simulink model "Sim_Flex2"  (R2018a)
settings: Solver=VariableStepAuto  StartTime=0.0  StopTime=20.0  RelTol=1e-3
InitFcn:
  | init
StopFcn:
  | pl
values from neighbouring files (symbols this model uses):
  d2r = 1/r2d    (= 0.0174532925199)    [init.m]
undefined symbols (not defined in the file or in its folder): Af, Ap, Bf, Bp, Cf, Cp, Df, Dp, TVC

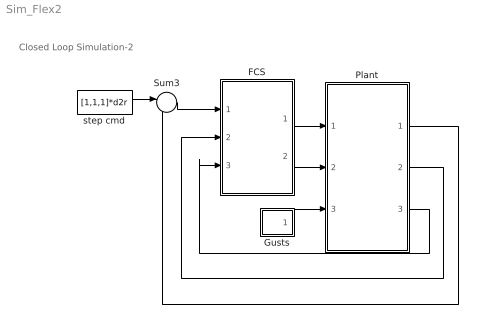
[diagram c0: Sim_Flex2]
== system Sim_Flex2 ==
  note: Closed Loop Simulation-2
  FCS : Subsystem
  Gusts : Subsystem
  Plant : Subsystem
  Sum3 : Sum  Inputs=|-+
  step cmd : Constant  Value=[1,1,1]*d2r
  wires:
  FCS/1(DY) -> Plant/1(Dy)
  FCS/2(DZ) -> Plant/2(Dz)
  Plant/3(NZY) -> FCS/3(Nzy)
  Plant/2(rate) -> FCS/2(pqr)
  Sum3/1 -> FCS/1(Attit)
  Plant/1(attit) -> Sum3/2
  step cmd/1 -> Sum3/1
  Gusts/1(Wgst) -> Plant/3(Gust)

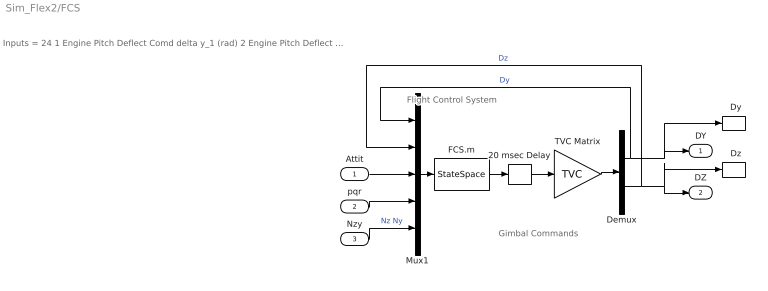
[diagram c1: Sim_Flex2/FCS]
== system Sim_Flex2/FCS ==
  note: Gimbal Commands
  note: Flight Control System
  note: Inputs = 24 1 Engine Pitch Deflect Comd delta y_1 (rad) 2 Engine Pitch Deflect Comd delta y_2 (rad) 3 Engine Pitch Deflect Comd delta y_3 (rad) 4 Engine Pitch Deflect Comd delta y_4 (rad) 5 Engine Pitch Deflect Comd delta y_5 (rad) 6 Engine Pitch Deflect Comd delta y_6 (rad) 7 Engine Pitch Deflect Comd delta y_7 (rad) 8 Engine Pitch Deflect Comd delta y_8 (rad) 9 Engine Yaw Deflect Commnd delta z_1 (rad) 10 Engine Yaw Deflect Commnd delta z_2 (rad) 11 Engine Yaw Deflect Commnd delta z_3 (rad) 12 Engine Yaw Deflect Commnd delta z_4 (rad) 13 Engine Yaw Deflect Commnd delta z_5 (rad) 14 Engine Yaw Deflect Commnd delta z_6 (rad) 15 Engine Yaw Deflect Commnd delta z_7 (rad) 16 Engine Yaw Deflect Commnd delta z_8 (rad) 17 Roll Attitude Error (rad) 18 Pitch Attitude Error (rad) 19 Yaw Attitude Error (rad) 20 Roll Rate (rad/sec) 21 Pitch Rate (rad/sec) 22 Yaw Rate (rad/sec) 23 Normal Acceleration NZ (ft/sec^2) 24 Lateral Acceleration NY (ft/sec^2)
  Attit : Inport
  pqr : Inport  Port=2
  Nzy : Inport  Port=3
  "  Dy" : ToWorkspace  VariableName=DY  SampleTime=-1
  "  Dz" : ToWorkspace  VariableName=DZ  SampleTime=-1
  20 msec Delay : TransportDelay  DelayTime="[1  1  1]*0.02"  InitialOutput="[0  0  0]"  PadeOrder=2
  Demux : Demux  Outputs=[8, 8]
  FCS.m : StateSpace  A=Af  B=Bf  C=Cf  D=Df  InitialCondition=0
  Mux1 : Mux  Inputs=[8, 8, 3, 3, 2]
  TVC Matrix : Gain  Gain=TVC  Multiplication=Matrix(K*u)
  DY : Outport
  DZ : Outport  Port=2
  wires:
  Demux/1 -> Mux1/1, "  Dy"/1, DY/1  "Dy"
  Demux/2 -> DZ/1, "  Dz"/1, Mux1/2  "Dz"
  Nzy/1 -> Mux1/5  "Nz Ny"
  Attit/1 -> Mux1/3
  pqr/1 -> Mux1/4
  Mux1/1 -> FCS.m/1
  TVC Matrix/1 -> Demux/1
  FCS.m/1 -> 20 msec Delay/1
  20 msec Delay/1 -> TVC Matrix/1

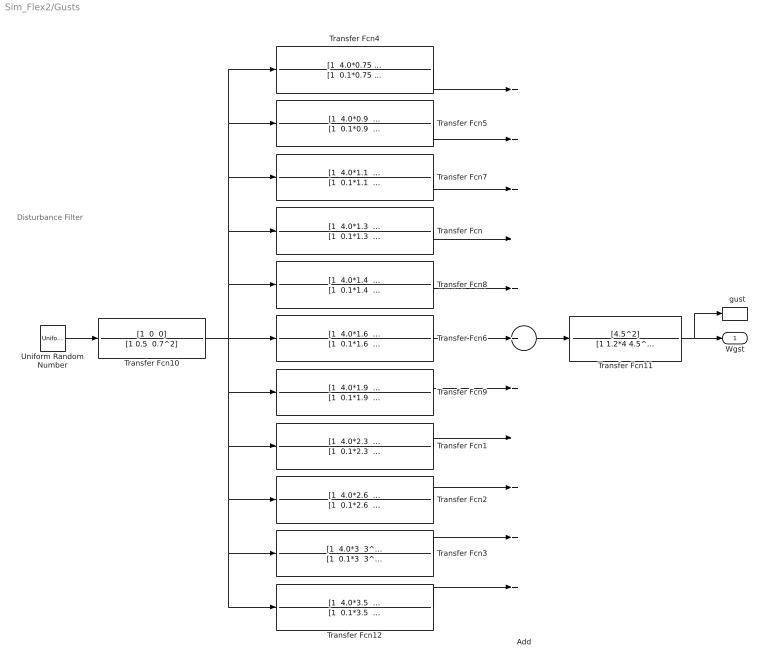
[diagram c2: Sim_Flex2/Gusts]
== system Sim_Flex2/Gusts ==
  note: Disturbance Filter
  "  gust" : ToWorkspace  VariableName=Wgst  SampleTime=-1
  Add : Sum  Inputs=+++++++++++
  Transfer Fcn : TransferFcn  Numerator="[1  4.0*1.3  1.3^2]"  Denominator="[1  0.1*1.3  1.3^2]"
  Transfer Fcn1 : TransferFcn  Numerator="[1  4.0*2.3  2.3^2]"  Denominator="[1  0.1*2.3  2.3^2]"
  Transfer Fcn10 : TransferFcn  Numerator="[1  0  0]"  Denominator="[1 0.5  0.7^2]"
  Transfer Fcn11 : TransferFcn  Numerator=[4.5^2]  Denominator=[1 1.2*4 4.5^2]
  Transfer Fcn12 : TransferFcn  Numerator="[1  4.0*3.5  3.5^2]"  Denominator="[1  0.1*3.5  3.5^2]"
  Transfer Fcn2 : TransferFcn  Numerator="[1  4.0*2.6  2.6^2]"  Denominator="[1  0.1*2.6  2.6^2]"
  Transfer Fcn3 : TransferFcn  Numerator="[1  4.0*3  3^2]"  Denominator="[1  0.1*3  3^2]"
  Transfer Fcn4 : TransferFcn  Numerator="[1  4.0*0.75  0.75^2]"  Denominator="[1  0.1*0.75  0.75^2]"
  Transfer Fcn5 : TransferFcn  Numerator="[1  4.0*0.9  0.9^2]"  Denominator="[1  0.1*0.9  0.9^2]"
  Transfer Fcn6 : TransferFcn  Numerator="[1  4.0*1.6  1.6^2]"  Denominator="[1  0.1*1.6  1.6^2]"
  Transfer Fcn7 : TransferFcn  Numerator="[1  4.0*1.1  1.1^2]"  Denominator="[1  0.1*1.1  1.1^2]"
  Transfer Fcn8 : TransferFcn  Numerator="[1  4.0*1.4  1.4^2]"  Denominator="[1  0.1*1.4  1.4^2]"
  Transfer Fcn9 : TransferFcn  Numerator="[1  4.0*1.9  1.9^2]"  Denominator="[1  0.1*1.9  1.9^2]"
  Uniform Random Number : UniformRandomNumber  SampleTime=0.1
  Wgst : Outport
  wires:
  Uniform Random Number/1 -> Transfer Fcn10/1
  Transfer Fcn12/1 -> Add/11
  Transfer Fcn3/1 -> Add/10
  Transfer Fcn11/1 -> "  gust"/1, Wgst/1
  Transfer Fcn6/1 -> Add/6
  Transfer Fcn5/1 -> Add/2
  Transfer Fcn4/1 -> Add/1
  Transfer Fcn/1 -> Add/4
  Add/1 -> Transfer Fcn11/1
  Transfer Fcn7/1 -> Add/3
  Transfer Fcn1/1 -> Add/8
  Transfer Fcn10/1 -> Transfer Fcn6/1, Transfer Fcn5/1, Transfer Fcn4/1, Transfer Fcn7/1, Transfer Fcn/1, Transfer Fcn8/1, Transfer Fcn1/1, Transfer Fcn2/1, Transfer Fcn12/1, Transfer Fcn3/1, Transfer Fcn9/1
  Transfer Fcn2/1 -> Add/9
  Transfer Fcn8/1 -> Add/5
  Transfer Fcn9/1 -> Add/7

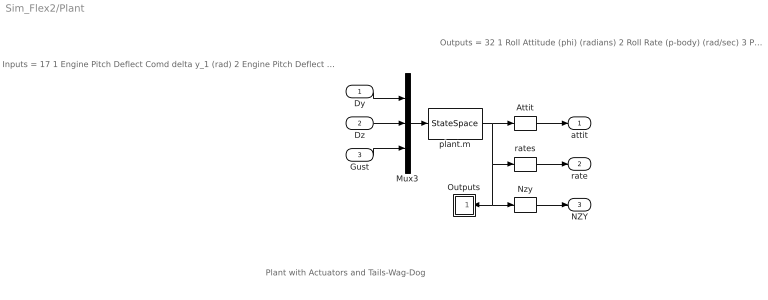
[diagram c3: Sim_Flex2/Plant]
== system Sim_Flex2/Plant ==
  note: Inputs = 17 1 Engine Pitch Deflect Comd delta y_1 (rad) 2 Engine Pitch Deflect Comd delta y_2 (rad) 3 Engine Pitch Deflect Comd delta y_3 (rad) 4 Engine Pitch Deflect Comd delta y_4 (rad) 5 Engine Pitch Deflect Comd delta y_5 (rad) 6 Engine Pitch Deflect Comd delta y_6 (rad) 7 Engine Pitch Deflect Comd delta y_7 (rad) 8 Engine Pitch Deflect Comd delta y_8 (rad) 9 Engine Yaw Deflect Commnd delta z_1 (rad) 10 Engine Yaw Deflect Commnd delta z_2 (rad) 11 Engine Yaw Deflect Commnd delta z_3 (rad) 12 Engine Yaw Deflect Commnd delta z_4 (rad) 13 Engine Yaw Deflect Commnd delta z_5 (rad) 14 Engine Yaw Deflect Commnd delta z_6 (rad) 15 Engine Yaw Deflect Commnd delta z_7 (rad) 16 Engine Yaw Deflect Commnd delta z_8 (rad) 17 Wind-Gust Velocity (ft/sec)
  note: Outputs = 32 1 Roll Attitude (phi) (radians) 2 Roll Rate (p-body) (rad/sec) 3 Pitch Attitude (thet) (radians) 4 Pitch Rate (q-body) (rad/sec) 5 Yaw Attitude (psi) (radians) 6 Yaw Rate (r-body) (rad/sec) 7 Angle of attack, alfa, (radian) 8 Angle of sideslip, beta, (radian) 9 Change in Altitude, delta-h, (feet) 10 Forward Acceleration (V-dot) (ft/sec) 11 Cross Range Velocity (Vcr) (ft/sec) 12 Rate-Gyro # 1, Roll Rate (Body) (rad/sec) 13 Rate-Gyro # 2, Pitch Rate (Body) (rad/sec) 14 Rate-Gyro # 3, Yaw Rate (Body) (rad/sec) 15 Accelerom # 1, (along Y), (ft/sec^2) Translat. Accelerat. 16 Accelerom # 2, (along Z), (ft/sec^2) Translat. Accelerat. 17 Engine #1 Pitch Deflection dy-1 (rad) 18 Engine #2 Pitch Deflection dy-2 (rad) 19 Engine #3 Pitch Deflection dy-3 (rad) 20 Engine #4 Pitch Deflection dy-4 (rad) 21 Engine #5 Pitch Deflection dy-5 (rad) 22 Engine #6 Pitch Deflection dy-6 (rad) 23 Engine #7 Pitch Deflection dy-7 (rad) 24 Engine #8 Pitch Deflection dy-8 (rad) 25 Engine #1 Yaw Deflection dz-1 (rad) 26 Engine #2 Yaw Deflection dz-2 (rad) 27 Engine #3 Yaw Deflection dz-3 (rad) 28 Engine #4 Yaw Deflection dz-4 (rad) 29 Engine #5 Yaw Deflection dz-5 (rad) 30 Engine #6 Yaw Deflection dz-6 (rad) 31 Engine #7 Yaw Deflection dz-7 (rad) 32 Engine #8 Yaw Deflection dz-8 (rad)
  note: Plant with Actuators and Tails-Wag-Dog
  Dy : Inport
  Dz : Inport  Port=2
  Gust : Inport  Port=3
  Attit : Selector  InputPortWidth=32  IndexOptions=Index vector (dialog)  Indices=[1,3,5]  OutputSizes=1
  Mux3 : Mux  Inputs=[8, 8, 1]
  Nzy : Selector  InputPortWidth=32  IndexOptions=Index vector (dialog)  Indices=[16,15]  OutputSizes=1
  Outputs : Subsystem
  plant.m : StateSpace  A=Ap  B=Bp  C=Cp  D=Dp  InitialCondition=0
  rates : Selector  InputPortWidth=32  IndexOptions=Index vector (dialog)  Indices=[12,13,14]  OutputSizes=1
  attit : Outport
  rate : Outport  Port=2
  NZY : Outport  Port=3
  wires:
  Nzy/1 -> NZY/1
  Gust/1 -> Mux3/3
  Attit/1 -> attit/1
  Mux3/1 -> plant.m/1
  plant.m/1 -> Outputs/1(in), Nzy/1, rates/1, Attit/1
  rates/1 -> rate/1
  Dz/1 -> Mux3/2
  Dy/1 -> Mux3/1

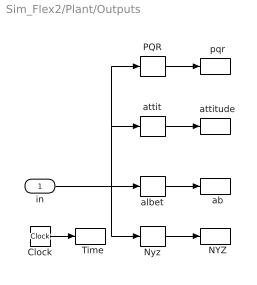
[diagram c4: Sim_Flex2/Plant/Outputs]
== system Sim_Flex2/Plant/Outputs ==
  in : Inport
  "  NYZ" : ToWorkspace  VariableName=Nyz  SampleTime=-1
  "  Time" : ToWorkspace  VariableName=tim  SampleTime=-1
  "  ab" : ToWorkspace  VariableName=albet  SampleTime=-1
  "  attitude" : ToWorkspace  VariableName=atti  SampleTime=-1
  "  pqr" : ToWorkspace  VariableName=pqr  SampleTime=-1
  Clock : Clock
  Nyz : Selector  InputPortWidth=32  IndexOptions=Index vector (dialog)  Indices=[15,16]  OutputSizes=1
  PQR : Selector  InputPortWidth=32  IndexOptions=Index vector (dialog)  Indices=[12, 13, 14]  OutputSizes=1
  albet : Selector  InputPortWidth=32  IndexOptions=Index vector (dialog)  Indices=[7,8]  OutputSizes=1
  attit : Selector  InputPortWidth=32  IndexOptions=Index vector (dialog)  Indices="[1  3   5]"  OutputSizes=1
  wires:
  Nyz/1 -> "  NYZ"/1
  in/1 -> PQR/1, attit/1, Nyz/1, albet/1
  attit/1 -> "  attitude"/1
  albet/1 -> "  ab"/1
  Clock/1 -> "  Time"/1
  PQR/1 -> "  pqr"/1
